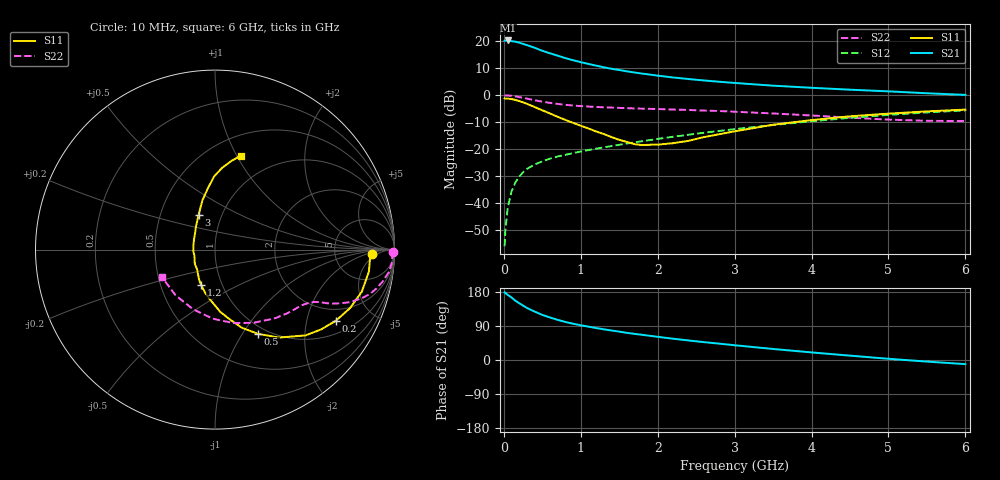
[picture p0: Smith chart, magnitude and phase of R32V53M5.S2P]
! SIEMENS Small Signal Semiconductors
! BFR181
! Si NPN RF Bipolar Junction Transistor in SOT23
! VCE = 2.5 V  IC = 3.5 mA
! Common Emitter S-Parameters:  May  1996
# GHz  S  MA  R  50
!  f  S11  S21  S12  S22
! GHz  MAG  ANG  MAG  ANG  MAG  ANG  MAG  ANG
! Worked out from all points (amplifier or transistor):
!   36 points, 10 MHz to 6 GHz, reference 50 ohm
!   highest |S21| = 20.3 dB at 50 MHz (marker M1)
!   |S21| within 3 dB of that: start of sweep to 426 MHz
!   unconditionally stable (mu >= 1): 1.275 GHz to 3.119 GHz
!   at 250 MHz: K = 0.34, MSG = 23.8 dB, |S12| = -28.5 dB
!   at 1.4 GHz: K = 1.03, MAG = 13.3 dB, |S12| = -18.8 dB
!   at 6 GHz: K = 0.86, MSG = 2.9 dB, |S12| = -5.6 dB
!   S11 on the Smith chart (normalised r, x): 10 MHz: 15, -3; 200 MHz: 1.48, -3.00; 500 MHz: 0.90, -1.17; 1.2 GHz: 0.80, -0.33; 3 GHz: 0.78, +0.32; 6 GHz: 0.70, +1.04
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0.01  0.8756 -1.5  10.25 178.5  0.0016 88.3  0.9943 -0.8
0.02  0.8649 -3.2  10.26 176.6  0.0032 90.1  0.9879 -1.5
0.05  0.8663 -8.1  10.37 172.1  0.0082 87.2  0.9899 -3.8
0.15  0.8196 -23.5  9.846 156.4  0.0242 76.7  0.9518 -10.7
0.2  0.7813 -30.5  9.43 149.9  0.031 73.2  0.9244 -13.6
0.25  0.7395 -37.0  8.943 143.5  0.0375 69.7  0.8978 -16.0
0.3  0.6946 -43.5  8.494 137.4  0.0431 68.3  0.8667 -18.0
0.4  0.6059 -54.0  7.592 127.8  0.0522 64.3  0.809 -21.2
0.5  0.5267 -63.0  6.665 119.0  0.0596 62.2  0.7598 -23.2
0.6  0.4606 -71.0  5.99 112.2  0.0671 60.3  0.7227 -24.6
0.7  0.3983 -77.9  5.413 105.9  0.0734 59.9  0.6913 -25.6
0.8  0.3495 -85.0  4.88 100.4  0.0788 59.1  0.6656 -26.3
0.9  0.3081 -90.5  4.459 95.7  0.0848 59.3  0.6456 -26.9
1.1  0.2426 -103.8  3.808 88.0  0.0965 59.8  0.6178 -28.3
1.2  0.2133 -110.9  3.54 84.2  0.1026 60.0  0.6076 -29.1
1.6  0.1367 -145.5  2.773 71.6  0.1275 60.7  0.5772 -32.3
2.2  0.1294 155.2  2.137 56.2  0.1704 60.6  0.5444 -39.2
3  0.2151 115.1  1.692 38.9  0.2357 57.2  0.4958 -51.6
3.5  0.2844 104.2  1.506 29.1  0.2813 53.7  0.4606 -62.3
4.5  0.4077 90.7  1.269 11.5  0.3818 44.0  0.3849 -92.0
5.5  0.5027 79.5  1.09 -4.2  0.4811 31.4  0.3363 -130.9
6  0.5425 74.6  1.016 -10.9  0.526 24.2  0.3329 -152.2
